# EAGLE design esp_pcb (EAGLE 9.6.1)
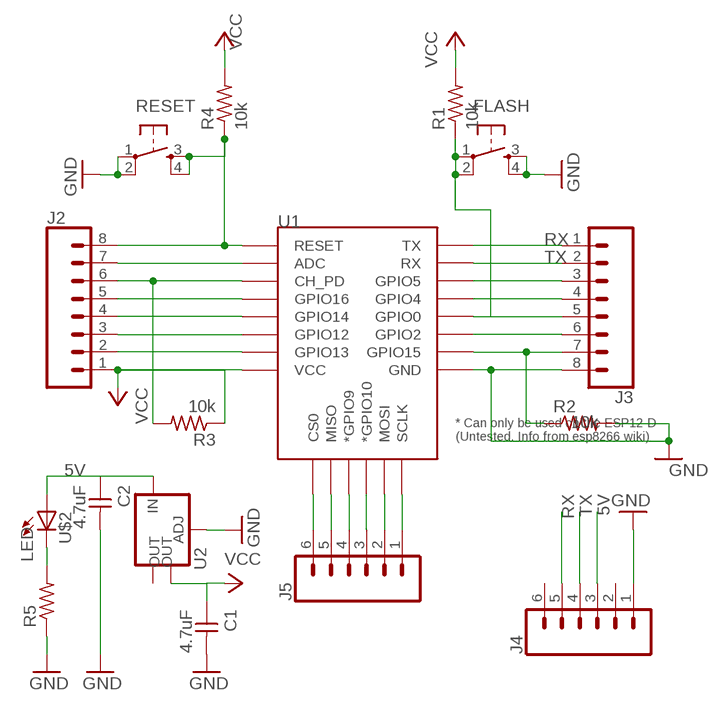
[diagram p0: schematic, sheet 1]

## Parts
C1  4.7uF  CAP-UNPOLARIZEDFAB  [C1206FAB]
C2  4.7uF  CAP-UNPOLARIZEDFAB  [C1206FAB]
FLASH  6MM_SWITCH6MM_SWITCH  [6MM_SWITCH]
J2  CONN_08"  [1X08]
J3  CONN_08"  [1X08]
J4  CONN_06SILK_FEMALE_PTH  [1X06]
J5  CONN_06SILK_FEMALE_PTH  [1X06]
R1  10k  RES-US1206FAB  [R1206FAB]
R2  10k  RES-US1206FAB  [R1206FAB]
R3  10k  RES-US1206FAB  [R1206FAB]
R4  10k  RES-US1206FAB  [R1206FAB]
R5  RES-US1206FAB  [R1206FAB]
RESET  6MM_SWITCH6MM_SWITCH  [6MM_SWITCH]
U1  ESP12ESMD  [ESP12E-SMD]
U2  V_REG_LM1117SOT223  [SOT223]
U$2  LED  LEDFAB1206  [LED1206FAB]

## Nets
5V: C2.1 J4.3 U2.3(IN) U$2.1(A)
GND: C1.2 C2.2 FLASH.3(S) FLASH.4(S1) J3.8 J4.1 R2.2 R5.1 RESET.1(P) RESET.2(P1) U1.GND U2.1(ADJ)
N$1: J5.6 U1.CS0
N$2: J5.5 U1.MISO
N$3: J5.4 U1.GPIO9(*GPIO9)
N$4: J5.3 U1.GPIO10(*GPIO10)
N$5: J5.2 U1.MOSI
N$6: J5.1 U1.SCLK
N$7: FLASH.1(P) FLASH.2(P1) J3.5 R1.1 U1.GPIO0
N$9: J3.3 U1.GPIO5
N$10: J3.4 U1.GPIO4
N$12: J3.6 U1.GPIO2
N$13: J3.7 R2.1 U1.GPIO15
N$14: J2.5 U1.GPIO16
N$15: J2.8 R4.1 RESET.3(S) RESET.4(S1) U1.RESET
N$16: J2.7 U1.ADC
N$17: J2.6 R3.2 U1.CH_PD
N$18: J2.4 U1.GPIO14
N$19: R5.2 U$2.2(C)
N$20: J2.3 U1.GPIO12
N$21: J2.2 U1.GPIO13
RX: J3.1 J4.5 U1.TXD0(TX)
TX: J3.2 J4.4 U1.RXD0(RX)
VCC: C1.1 J2.1 R1.2 R3.1 R4.2 U1.VCC U2.4(OUT)
Unconnected: J4.2 J4.6 U2.2(OUT)

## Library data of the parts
C1 C2 = fab:CAP-UNPOLARIZED
FLASH RESET = fab:6MM_SWITCH: OMRON SWITCH
J2 J3 = SparkFun-Connectors:CONN_08: Multi connection point. Often used as Generic Header-pin footprint for 0.1 inch spaced/style header connections On any of the 0.1 inch spaced packages, you can populate with these: Break Away Headers - Straight (PRT-00116) Break Away Male Headers - Right Angle (PRT-00553) Female Headers (PRT-00115)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; PROD_ID: CONN-08438
J4 J5 = SparkFun-Connectors:CONN_06: Multi connection point. Often used as Generic Header-pin footprint for 0.1 inch spaced/style header connections On any of the 0.1 inch spaced packages, you can populate with these: Break Away Headers - Straight (PRT-00116) Break Away Male Headers - Right Angle (PRT-00553) Female Headers (PRT-00115)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; PROD_ID: CONN-08437
R1-R5 = fab:RES-US: Resistor (US Symbol)
U1 = esp8266modules:ESP12E: ESP12E Module
U2 = SparkFun-IC-Power:V_REG_LM1117: Voltage Regulator LM1117 Standard adjustable voltage regulator but in SMD form. Spark Fun Electronics SKU : COM-00595; PROD_ID: VREG-08170
U$2 = fab:LED: LED

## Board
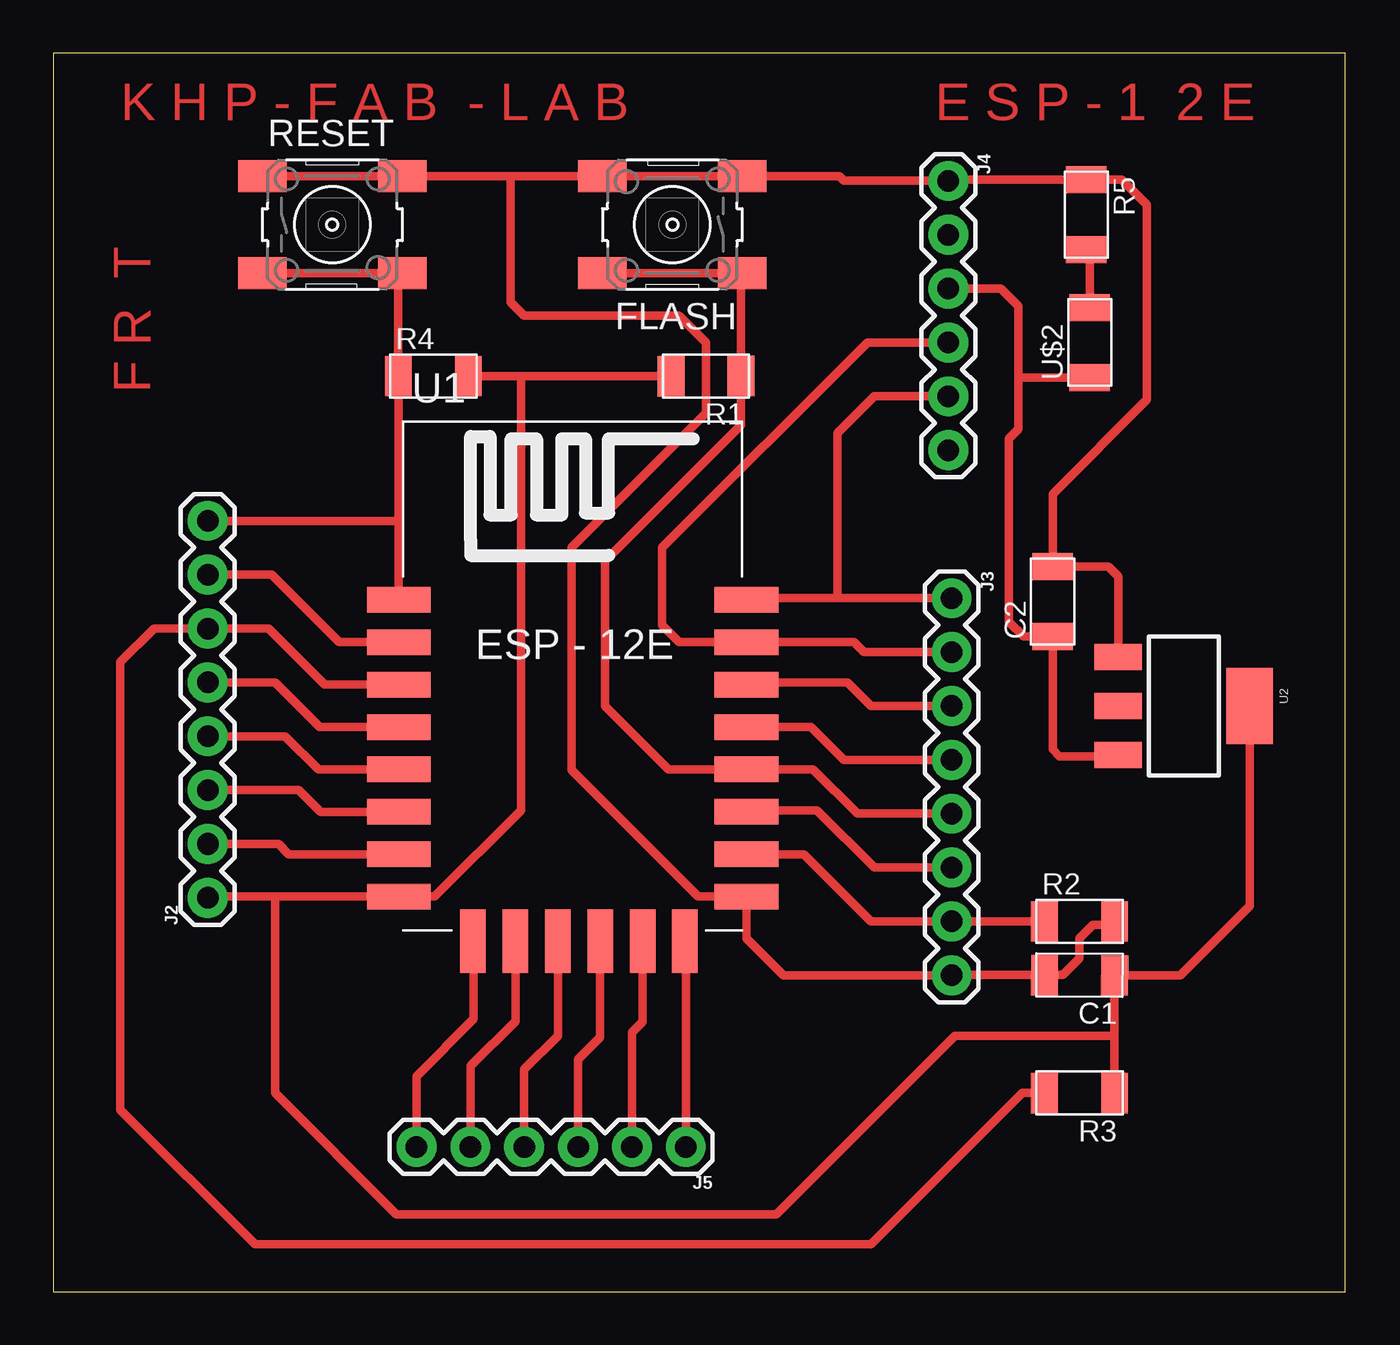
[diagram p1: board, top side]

Size 60.96 x 58.42 mm. Coordinates in mm from the lower left corner, seen from the top.
Outline: 0,0 60.96,0 60.96,58.42 0,58.42 0,0
Copper layers (1*16): Top 0.035mm / dielectric 1.5mm / Bottom 0.035mm
Design rules "default": minimum track width 10mil, minimum drill 24mil, track to track 8mil, track to pad 8mil, pad to pad 8mil, via to via 8mil, smd to smd 8mil, copper to edge 40mil, drill to drill 8mil, minimum pad ring 10mil, minimum via ring 8mil, stop-mask expansion 4mil, vias tented up to drill 0mil, thermal gap 10mil

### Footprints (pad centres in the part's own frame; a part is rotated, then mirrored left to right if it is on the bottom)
C1206FAB = smd 1.27 x 1.905: 1 -1.651,0; 2 1.651,0
6MM_SWITCH = smd 2.286 x 1.524: 1 -3.302,2.286; 2 3.302,2.286; 3 -3.302,-2.286; 4 3.302,-2.286
1X08 = drill 1.016 pad 1.88: 1 0,0; 2 2.54,0; 3 5.08,0; 4 7.62,0; 5 10.16,0; 6 12.7,0; 7 15.24,0; 8 17.78,0
1X06 = drill 1.016 pad 1.88: 1 0,0; 2 2.54,0; 3 5.08,0; 4 7.62,0; 5 10.16,0; 6 12.7,0
R1206FAB = smd 1.27 x 1.905: 1 -1.651,0; 2 1.651,0
ESP12E-SMD = smd 3 x 1.2: ADC -8.3,3.8; CH_PD -8.3,1.8; GND 8.1,-8.2; GPIO0 8.1,-2.2; GPIO2 8.1,-4.2; GPIO4 8.1,-0.2; GPIO5 8.1,1.8; GPIO12 -8.3,-4.2; GPIO13 -8.3,-6.2; GPIO14 -8.3,-2.2; GPIO15 8.1,-6.2; GPIO16 -8.3,-0.2; RESET -8.3,5.8; RXD0 8.1,3.8; TXD0 8.1,5.8; VCC -8.3,-8.2 | smd 1.2 x 3: CS0 -4.8,-10.3; GPIO9 -0.8,-10.3; GPIO10 1.2,-10.3; MISO -2.8,-10.3; MOSI 3.2,-10.3; SCLK 5.2,-10.3
SOT223 = smd 1.219 x 2.235: 1 -2.311,-3.099; 2 0,-3.099; 3 2.311,-3.099 | smd 3.6 x 2.2: 4 0,3.099
LED1206FAB = smd 1.27 x 1.905: 1 -1.651,0; 2 1.651,0

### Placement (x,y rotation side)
C1  48.42,14.92 179.8 top
C2  47.15,32.54 90 top
FLASH  29.21,50.32 180 top
J2  7.3,18.57 90 top
J3  42.39,32.7 270 top
J4  42.23,52.39 270 top
J5  29.84,6.83 180 top
R1  30.8,43.18 180.2 top
R2  48.42,17.46 0 top
R3  48.42,9.37 180 top
R4  17.94,43.18 0 top
R5  48.74,50.8 270 top
RESET  13.18,50.32 0 top
U1  24.61,26.83 0 top
U2  53.34,27.62 270 top
U$2  48.9,44.77 90 top

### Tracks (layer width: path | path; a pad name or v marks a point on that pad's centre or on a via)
5V
  Top 0.406: J4.3 44.7,47.31 45.53,46.48 45.53,43.12 | U$2.1 45.53,43.12 | 45.53,43.12 45.53,40.67 45.09,40.23 45.09,31.59 45.78,30.89 C2.1 47.15,25.56 47.47,25.24 50.17,25.24 U2.3
GND
  Top 0.406: RESET.1 RESET.2 21.59,52.61 | 21.59,52.61 FLASH.4 FLASH.3 37.08,52.61 37.31,52.39 J4.1 42.29,52.45 R5.1 50.42,52.45 51.59,51.28 51.59,42.07 47.15,37.62 C2.2 49.78,34.2 50.24,33.74 U2.1 | R2.2 49.91,17.3 49.05,17.3 48.42,16.67 48.42,15.72 47.63,14.93 C1.2 J3.8 34.45,14.92 32.71,16.66 U1.GND 30.43,18.63 24.45,24.61 24.45,35.08 30.8,41.43 30.8,44.77 29.53,46.04 22.23,46.04 21.59,46.67 21.59,52.61
N$1
  Top 0.406: J5.6 17.14,10.16 19.84,12.86 19.84,16.49 U1.CS0
N$2
  Top 0.406: J5.5 19.68,10.64 21.81,12.76 U1.MISO
N$3
  Top 0.406: J5.4 22.23,10.48 23.81,12.06 U1.GPIO9
N$4
  Top 0.406: J5.3 24.77,10.95 25.81,11.99 U1.GPIO10
N$5
  Top 0.406: J5.2 27.3,12.22 27.81,12.72 U1.MOSI
N$6
  Top 0.406: J5.1 29.84,16.49 U1.SCLK
N$7
  Top 0.406: FLASH.1 32.38,48.04 | 32.38,48.04 FLASH.2 | 32.38,48.04 32.45,47.97 R1.1 32.45,40.86 26.04,34.45 26.04,27.62 29.03,24.63 U1.GPIO0 35.85,24.63 37.94,22.54 J3.5
N$9
  Top 0.406: J3.3 38.58,27.62 37.47,28.73 32.81,28.73 U1.GPIO5
N$10
  Top 0.406: U1.GPIO4 35.76,26.63 37.31,25.08 J3.4
N$12
  Top 0.406: J3.6 38.73,20 36.04,22.7 32.78,22.7 U1.GPIO2
N$13
  Top 0.406: R2.1 J3.7 38.58,17.46 35.41,20.63 U1.GPIO15
N$14
  Top 0.406: J2.5 10.48,28.73 12.58,26.63 U1.GPIO16
N$15
  Top 0.406: U1.RESET 16.31,36.51 | 16.31,36.51 16.31,43.16 R4.1 16.29,47.85 RESET.4 RESET.3 | J2.8 16.15,36.35 16.31,36.51
N$16
  Top 0.406: U1.ADC 13.5,30.63 10.32,33.81 J2.7
N$17
  Top 0.406: U1.CH_PD 12.8,28.63 10.16,31.27 J2.6 4.76,31.27 3.17,29.69 3.17,8.57 9.53,2.22 38.58,2.22 45.72,9.37 R3.2
N$18
  Top 0.406: U1.GPIO14 12.52,24.63 10.95,26.19 J2.4
N$19
  Top 0.406: U$2.2 48.9,48.99 R5.2
N$20
  Top 0.406: J2.3 11.59,23.65 12.46,22.78 12.54,22.7 12.61,22.63 U1.GPIO12
N$21
  Top 0.406: U1.GPIO13 11.12,20.63 10.64,21.11 J2.2
RX
  Top 0.406: J3.1 36.99,32.7 | 36.99,32.7 32.78,32.7 U1.TXD0 | J4.5 38.73,42.23 36.99,40.48 36.99,32.7
TX
  Top 0.406: J3.2 38.26,30.16 37.78,30.64 U1.RXD0 29.54,30.63 28.73,31.43 28.73,35.08 38.42,44.77 J4.4
VCC
  Top 0.406: 10.48,18.63 U1.VCC 17.99,18.63 22.07,22.7 22.07,43.18 | 10.48,18.63 7.36,18.63 J2.1 | R4.2 22.07,43.18 | 22.07,43.18 R1.2 | R3.1 50.07,12.06 | 50.07,12.06 C1.1 | C1.1 | C1.1 53.17,14.92 56.44,18.18 U2.4 | 50.07,12.06 42.55,12.06 34.13,3.65 16.19,3.65 10.48,9.37 10.48,18.63

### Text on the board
Top: K H P - F A B - L A B | E S P - 1 2 E | F R T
